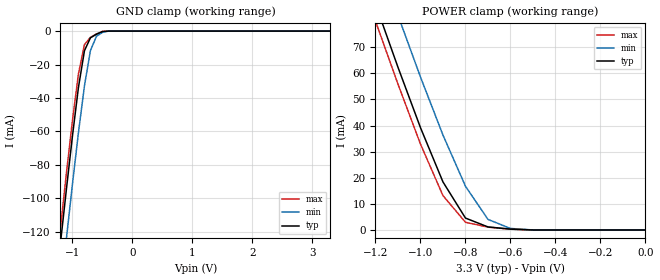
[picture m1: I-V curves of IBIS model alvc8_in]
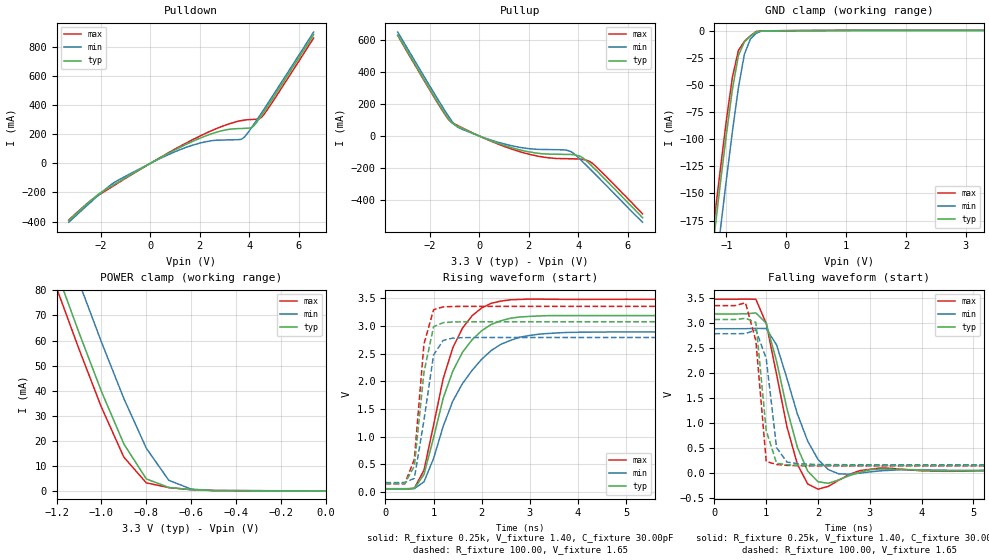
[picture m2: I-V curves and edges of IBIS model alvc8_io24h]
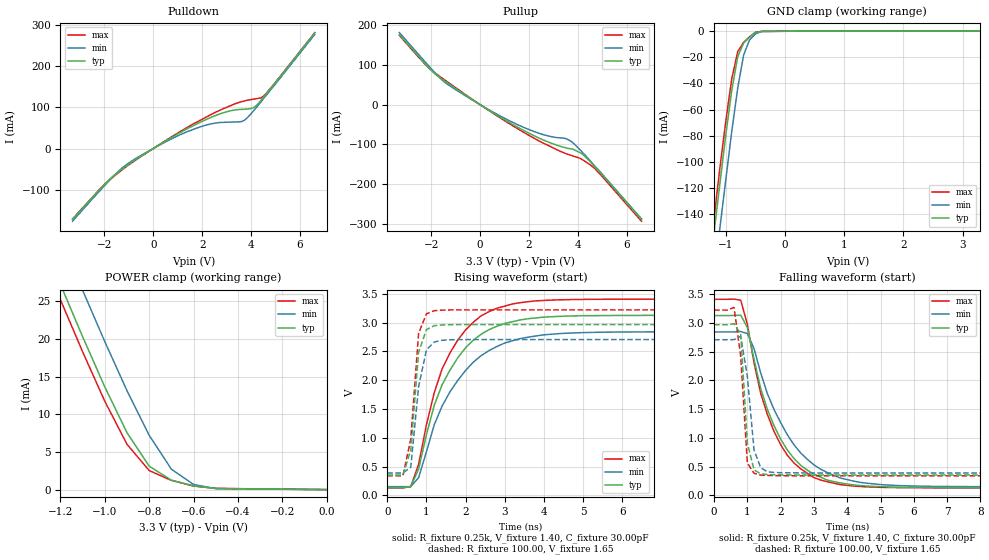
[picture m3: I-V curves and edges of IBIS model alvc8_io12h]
| IBIS file 162245ah.ibs created by s2ibis2 version 1.1
| North Carolina State University Electronics Research Laboratory  1995
[IBIS ver]   2.1
[File name]   162245ah.ibs
[File Rev]   1.0
[Date]   03/01/99 rtk rtk
[Source]   Integrated Device Technology, Inc.
[Notes]   1.Temperatures: typ=25C, min=100C, max=0C 2.RRmp rates based
   on 50 ohm load.
[Disclaimer] Integrated Device Technology, Inc. ("IDT") hereby grants the
   user of this IBIS model a non-exclusive, nontransferable
   license to use this IBIS model under the following terms. The
   user is granted this license only to use the IBIS model and is
   not granted rights to sell, copy (except as needed to run the
   IBIS model), rent, lease or sub-license the IBIS model in
   whole or in part, or in modified form to anyone. The User may
   modify the IBIS model to suit its specific applications, but
   rights to derivative works and such modifications shall belong
   to IDT. This IBIS model is provided on an AS IS" basis and IDT
   makes absolutely no warranty with respect to the information
   contained herein. IDT DISCLAIMS AND CUSTOMER WAIVES ALL
   WARRANTIES, EXPRESS AND IMPLIED, INCLUDING WARRANTIES OF
   MERCHANTABILITY AND FITNESS FOR A PARTICULAR PURPOSE. THE
   ENTIRE RISK AS TO QUALITY AND PERFORMANCE IS WITH THE USER
   ACCORDINGLY, IN NO EVENT SHALL IDT BE LIABLE FOR ANY DIRECT OR
   INDIRECT DAMAGES, WHETHER IN CONTRACT OR TORT, INCLUDING ANY
   LOST PROFITS OR OTHER INCIDENTAL, CONSEQUENTIAL, EXEMPLARY, OR
   PUNITIVE DAMAGES ARISING OUT OF THE USE OR APPLICATION OF THE
   IBIS model. Further, IDT reserves the right to make changes
   without notice to any product herein to improve reliability,
   function, or design. IDT does not convey any license under
   patent rights or any other intellectual property rights,
   including those of third parties. IDT is not obligated to
   provide maintenance or support for the licensed IBIS model.
[Copyright]   Copyright 1997, Integrated Device Technology, Inc. all rights
   reserved
|   Component ALVCH162245
[Component]   ALVCH162245
[Manufacturer]   Integrated Device Technology
[Package]
| PA48
| variable   typ   min   max
R_pkg   6.50m   5.00m   10.00m
L_pkg   3.20nH   2.50nH   4.40nH
C_pkg   0.27pF   0.01pF   0.98pF
| PV48   typ   min   max
|R_pkg   6.5m   5.00m   10.00m
|L_pkg   4.75nH   3.82nH   6.72nH
|C_pkg   0.24pF   0.01pF   1.55pF
[Pin]  signal_name   model_name   R_pin   L_pin   C_pin
1   1DIR   alvc8_in
2   1B1   alvc8_io24h
3   1B2   alvc8_io24h
4   GND   GND
5   1B3   alvc8_io24h
6   1B4   alvc8_io24h
7   VCC   POWER
8   1B5   alvc8_io24h
9   1B6   alvc8_io24h
10   GND   GND
11   1B7   alvc8_io24h
12   1B8   alvc8_io24h
13   2B1   alvc8_io24h
14   2B2   alvc8_io24h
15   GND   GND
16   2B3   alvc8_io24h
17   2B4   alvc8_io24h
18   VCC   POWER
19   2B5   alvc8_io24h
20   2B6   alvc8_io24h
21   GND   GND
22   2B7   alvc8_io24h
23   2B8   alvc8_io24h
24   2DIR   alvc8_in
25   2OEB   alvc8_in
26   2A8   alvc8_io12h
27   2A7   alvc8_io12h
28   GND   GND
29   2A6   alvc8_io12h
30   2A5   alvc8_io12h
31   VCC   POWER
32   2A4   alvc8_io12h
33   2A3   alvc8_io12h
34   GND   GND
35   2A2   alvc8_io12h
36   2A1   alvc8_io12h
37   1A8   alvc8_io12h
38   1A7   alvc8_io12h
39   GND   GND
40   1A6   alvc8_io12h
41   1A5   alvc8_io12h
42   VCC   POWER
43   1A4   alvc8_io12h
44   1A3   alvc8_io12h
45   GND   GND
46   1A2   alvc8_io12h
47   1A1   alvc8_io12h
48   1OEB   alvc8_in
| Models and submodels in the file (3): alvc8_in (Input), alvc8_io24h (I/O), alvc8_io12h (I/O)
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| in   in   dummy_model
| oe   oe   dummy_model
|   Model alvc8_in
[Model]   alvc8_in
Model_type   Input
Vinl =  0.800V
Vinh =  2.000V
C_comp   3.00pF   NA   NA
[Temperature Range]   25.00   100.00   0.000
[Voltage Range]   3.30V   3.00V   3.60V
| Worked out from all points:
|   GND clamp passes 1 mA (typ) near -0.54 V on its own axis
|   POWER clamp passes 1 mA (typ) near -0.68 V on its own axis
[GND_clamp]
| voltage   I(typ)   I(min)   I(max)
-3.3V     -860mA     -887mA     -851mA
-1.3V     -161mA     -190mA     -151mA
-1.2V     -127mA     -157mA     -118mA
-1.1V     -94.41mA   -124mA     -84.85mA
-1V       -62.78mA   -91.54mA   -53.52mA
-900mV    -33.71mA   -60.78mA   -25.6mA
-800mV    -11.74mA   -32.83mA   -8.09mA
-700mV    -4.033mA   -11.65mA   -3.7mA
-600mV    -1.899mA   -3.108mA   -1.699mA
-500mV    -308uA     -810uA     -172uA
-400mV    -3.848nA   -9.872uA   -399pA
3.3V      39.6pA     19.33nA    26.4pA
[POWER_clamp]
| voltage   I(typ)   I(min)   I(max)
-3.3V     630mA      648mA      624mA
-1.2V     86.56mA    106mA      80.02mA
-1.1V     62.33mA    82.22mA    55.88mA
-1V       39.2mA     58.61mA    32.91mA
-900mV    18.4mA     36.35mA    13.15mA
-800mV    4.556mA    16.76mA    2.954mA
-700mV    1.164mA    4.056mA    1.087mA
-600mV    320uA      578uA      299uA
-500mV    40.08nA    12.23uA    3.465nA
0V        39.6pA     59.11pA    43.2pA
|   Model alvc8_io24h
[Model]   alvc8_io24h
Model_type   I/O
Polarity   Non-Inverting
Enable   Active-High
Vinl =  0.000V
Vinh =  2.000V
Vmeas =  1.500V
C_comp   3.00pF   NA   NA
[Temperature Range]   25.00   100.00   0.000
[Voltage Range]   3.30V   3.00V   3.60V
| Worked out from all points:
|   slope of the pulldown table from 0 to 0.495 V, typ, clamps not added: 10.5 ohm
|   slope of the pullup table from 0 to 0.495 V, typ, clamps not added: 16.1 ohm
|   GND clamp passes 1 mA (typ) near -0.50 V on its own axis
|   POWER clamp passes 1 mA (typ) near -0.66 V on its own axis
|   rising waveform, R_fixture 0.25k, V_fixture 1.40, C_fixture 30.00pF: 20-80 % time 723ps typ, 920ps min, 623ps max; typ from 0.055 V to 3.19 V
|   rising waveform, R_fixture 100.00, V_fixture 1.65: 20-80 % time 248ps typ, 279ps min, 194ps max; typ from 0.155 V to 3.08 V
|   falling waveform, R_fixture 0.25k, V_fixture 1.40, C_fixture 30.00pF: 20-80 % time 444ps typ, 538ps min, 413ps max; typ from 3.19 V to 0.055 V
|   falling waveform, R_fixture 100.00, V_fixture 1.65: 20-80 % time 187ps typ, 176ps min, 171ps max; typ from 3.08 V to 0.155 V
[Pulldown]
| voltage   I(typ)   I(min)   I(max)
-3.3V     -392mA     -404mA     -389mA
-2.3V     -240mA     -249mA     -241mA
-1.5V     -149mA     -136mA     -156mA
300mV     28.8mA     25.5mA     30.3mA
1.4V      127mA      107mA      135mA
2.4V      199mA      153mA      219mA
3.6V      239mA      163mA      291mA
3.8V      240mA      180mA      297mA
4.2V      260mA      272mA      302mA
4.4V      306mA      322mA      306mA
4.6V      356mA      373mA      337mA
6.6V      883mA      901mA      860mA
[Pullup]
| voltage   I(typ)   I(min)   I(max)
-3.3V     630mA      649mA      628mA
-1.4V     142mA      160mA      137mA
-1.1V     80.6mA     90.7mA     83.6mA
-900mV    63mA       57.7mA     67.6mA
400mV     -25.1mA    -21.5mA    -27.4mA
1.6V      -85mA      -69.5mA    -95.9mA
2.6V      -111mA     -84mA      -132mA
3.4V      -115mA     -86.1mA    -141mA
3.7V      -115mA     -97.1mA    -142mA
4.1V      -128mA     -149mA     -144mA
4.5V      -179mA     -210mA     -162mA
6.6V      -510mA     -538mA     -486mA
[GND_clamp]
| voltage   I(typ)   I(min)   I(max)
-3.3V     -1.238A    -1.278A    -1.225A
-1.3V     -235mA     -278mA     -221mA
-1.2V     -187mA     -230mA     -173mA
-1.1V     -140mA     -183mA     -127mA
-1V       -95.39mA   -137mA     -82.2mA
-900mV    -54.08mA   -92.95mA   -42.96mA
-800mV    -22.96mA   -52.74mA   -18.28mA
-700mV    -10.43mA   -21.77mA   -9.816mA
-600mV    -5.251mA   -7.746mA   -4.745mA
-500mV    -1.015mA   -2.281mA   -688uA
-400mV    -144uA     -128uA     -169uA
3.3V      264uA      161uA      341uA
[POWER_clamp]
| voltage   I(typ)   I(min)   I(max)
-3.3V     638mA      656mA      632mA
-1.2V     87.67mA    108mA      81.05mA
-1.1V     63.19mA    83.28mA    56.62mA
-1V       39.75mA    59.43mA    33.41mA
-900mV    18.73mA    36.86mA    13.47mA
-800mV    4.8mA      17.05mA    3.222mA
-700mV    1.374mA    4.243mA    1.32mA
-600mV    498uA      728uA      497uA
-500mV    146uA      134uA      162uA
0V        111pA      156pA      121pA
[Ramp]
| variable   typ   min   max
dV/dt_r   1.48/0.31n   1.29/0.30n   1.66/0.22n
dV/dt_f   1.63/0.28n   1.45/0.31n   1.80/0.19n
R_load = 50.00
[Rising Waveform]
R_fixture = 0.25k
V_fixture = 1.40
C_fixture = 30.00pF
R_dut = 7.00m
L_dut = 3.30nH
C_dut = 0.29pF
| time   V(typ)   V(min)   V(max)
0s        55.43mV    62mV       53.03mV
600ps     66.6mV     63.52mV    70.73mV
800ps     318mV      185mV      393mV
1ns       982mV      608mV      1.211V
1.2ns     1.697V     1.189V     2.05V
1.4ns     2.186V     1.644V     2.606V
1.8ns     2.751V     2.198V     3.185V
2.4ns     3.095V     2.67V      3.451V
3.8ns     3.189V     2.885V     3.481V
19.8ns    3.189V     2.893V     3.482V
[Rising Waveform]
R_fixture = 100.00
V_fixture = 1.65
R_dut = 7.00m
L_dut = 3.30nH
C_dut = 0.29pF
| time   V(typ)   V(min)   V(max)
0s        155mV      172mV      148mV
400ps     155mV      173mV      148mV
600ps     469mV      249mV      594mV
800ps     2.166V     1.299V     2.675V
1ns       2.988V     2.477V     3.294V
1.2ns     3.061V     2.741V     3.346V
1.4ns     3.073V     2.782V     3.353V
2ns       3.077V     2.793V     3.355V
19.8ns    3.077V     2.793V     3.355V
[Falling Waveform]
R_fixture = 0.25k
V_fixture = 1.40
C_fixture = 30.00pF
R_dut = 7.00m
L_dut = 3.30nH
C_dut = 0.29pF
| time   V(typ)   V(min)   V(max)
0s        3.189V     2.893V     3.482V
800ps     3.208V     2.901V     3.481V
1ns       3.002V     2.896V     2.998V
1.2ns     2.239V     2.568V     1.977V
1.4ns     1.294V     1.899V     934mV
1.6ns     525mV      1.193V     186mV
2ns       -168mV     277mV      -316mV
2.4ns     -131mV     -10.2mV    -138mV
3.2ns     86.4mV     50.55mV    107mV
19.8ns    55.43mV    62mV       53.03mV
[Falling Waveform]
R_fixture = 100.00
V_fixture = 1.65
R_dut = 7.00m
L_dut = 3.30nH
C_dut = 0.29pF
| time   V(typ)   V(min)   V(max)
0s        3.077V     2.793V     3.355V
400ps     3.077V     2.793V     3.355V
600ps     3.101V     2.795V     3.411V
800ps     3.02V      2.869V     2.651V
1ns       857mV      2.294V     237mV
1.2ns     202mV      512mV      177mV
1.4ns     172mV      227mV      160mV
1.6ns     163mV      194mV      154mV
2ns       157mV      178mV      149mV
19.8ns    155mV      172mV      148mV
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|   Model alvc8_io12h
[Model]   alvc8_io12h
Model_type   I/O
Polarity   Non-Inverting
Enable   Active-High
Vinl =  0.000V
Vinh =  2.000V
Vmeas =  1.500V
C_comp   3.00pF   NA   NA
[Temperature Range]   25.00   100.00   0.000
[Voltage Range]   3.30V   3.00V   3.60V
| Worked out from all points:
|   slope of the pulldown table from 0 to 0.495 V, typ, clamps not added: 27.5 ohm
|   slope of the pullup table from 0 to 0.495 V, typ, clamps not added: 25.8 ohm
|   GND clamp passes 1 mA (typ) near -0.50 V on its own axis
|   POWER clamp passes 1 mA (typ) near -0.67 V on its own axis
|   rising waveform, R_fixture 0.25k, V_fixture 1.40, C_fixture 30.00pF: 20-80 % time 1.07ns typ, 1.21ns min, 991ps max; typ from 0.137 V to 3.12 V
|   rising waveform, R_fixture 100.00, V_fixture 1.65: 20-80 % time 184ps typ, 259ps min, 200ps max; typ from 0.354 V to 2.96 V
|   falling waveform, R_fixture 0.25k, V_fixture 1.40, C_fixture 30.00pF: 20-80 % time 1.13ns typ, 1.37ns min, 1.04ns max; typ from 3.12 V to 0.137 V
|   falling waveform, R_fixture 100.00, V_fixture 1.65: 20-80 % time 176ps typ, 241ps min, 216ps max; typ from 2.96 V to 0.354 V
[Pulldown]
| voltage   I(typ)   I(min)   I(max)
-3.3V     -172mA     -177mA     -171mA
-1.8V     -76mA      -78.1mA    -76.9mA
-1.3V     -51.4mA    -48.7mA    -53mA
-700mV    -26.3mA    -23.6mA    -27.4mA
800mV     28.7mA     25.1mA     30.3mA
1.8V      60.3mA     50.2mA     64.7mA
2.9V      87.5mA     63.7mA     97.9mA
3.7V      95.5mA     67.7mA     115mA
4.1V      99.3mA     91.8mA     120mA
4.5V      124mA      121mA      127mA
5V        161mA      157mA      161mA
6.6V      281mA      277mA      282mA
[Pullup]
| voltage   I(typ)   I(min)   I(max)
-3.3V     176mA      181mA      174mA
-1.9V     80.3mA     83.6mA     82mA
-1.5V     61.8mA     58.9mA     64.3mA
-1V       40.8mA     37.7mA     42.5mA
400mV     -15.6mA    -14.2mA    -16.4mA
1.7V      -62.2mA    -54.9mA    -66.6mA
2.9V      -96.6mA    -80.2mA    -106mA
3.5V      -108mA     -85.3mA    -123mA
3.8V      -112mA     -96mA      -129mA
4.2V      -125mA     -121mA     -139mA
4.7V      -156mA     -155mA     -161mA
6.6V      -289mA     -287mA     -293mA
[GND_clamp]
| voltage   I(typ)   I(min)   I(max)
-3.3V     -1.019A    -1.052A    -1.008A
-1.3V     -194mA     -229mA     -182mA
-1.2V     -154mA     -189mA     -143mA
-1.1V     -116mA     -150mA     -104mA
-1V       -78.66mA   -113mA     -68.13mA
-900mV    -44.91mA   -76.33mA   -36.12mA
-800mV    -19.38mA   -43.36mA   -15.48mA
-700mV    -9.002mA   -18.09mA   -8.455mA
-600mV    -4.636mA   -6.615mA   -4.212mA
-500mV    -941uA     -2.052mA   -652uA
-400mV    -144uA     -128uA     -169uA
3.3V      264uA      161uA      341uA
[POWER_clamp]
| voltage   I(typ)   I(min)   I(max)
-3.3V     183mA      189mA      181mA
-1.3V     34.33mA    40.55mA    32.29mA
-1.2V     27.22mA    33.44mA    25.19mA
-1.1V     20.28mA    26.44mA    18.28mA
-1V       13.61mA    19.62mA    11.71mA
-900mV    7.542mA    13.11mA    6.005mA
-800mV    3.103mA    7.194mA    2.527mA
-700mV    1.249mA    2.702mA    1.219mA
-600mV    484uA      674uA      476uA
-500mV    146uA      134uA      162uA
0V        111pA      156pA      121pA
[Ramp]
| variable   typ   min   max
dV/dt_r   1.29/0.24n   1.13/0.30n   1.44/0.25n
dV/dt_f   1.26/0.26n   1.08/0.26n   1.40/0.24n
R_load = 50.00
[Rising Waveform]
R_fixture = 0.25k
V_fixture = 1.40
C_fixture = 30.00pF
R_dut = 7.00m
L_dut = 3.30nH
C_dut = 0.29pF
| time   V(typ)   V(min)   V(max)
0s        137mV      152mV      131mV
600ps     152mV      153mV      153mV
800ps     459mV      307mV      538mV
1.2ns     1.566V     1.227V     1.783V
1.4ns     1.921V     1.551V     2.196V
1.8ns     2.389V     1.996V     2.696V
2.4ns     2.799V     2.427V     3.119V
3.2ns     3.016V     2.685V     3.324V
5.6ns     3.122V     2.834V     3.405V
19.8ns    3.125V     2.84V      3.407V
[Rising Waveform]
R_fixture = 100.00
V_fixture = 1.65
R_dut = 7.00m
L_dut = 3.30nH
C_dut = 0.29pF
| time   V(typ)   V(min)   V(max)
0s        354mV      389mV      341mV
400ps     354mV      390mV      341mV
600ps     788mV      488mV      976mV
800ps     2.487V     1.886V     2.814V
1ns       2.877V     2.527V     3.153V
1.2ns     2.947V     2.663V     3.206V
1.4ns     2.959V     2.693V     3.216V
2ns       2.965V     2.705V     3.22V
19.8ns    2.965V     2.705V     3.22V
[Falling Waveform]
R_fixture = 0.25k
V_fixture = 1.40
C_fixture = 30.00pF
R_dut = 7.00m
L_dut = 3.30nH
C_dut = 0.29pF
| time   V(typ)   V(min)   V(max)
0s        3.125V     2.84V      3.407V
800ps     3.131V     2.846V     3.392V
1ns       2.917V     2.813V     2.972V
1.4ns     1.855V     2.128V     1.774V
1.8ns     1.213V     1.493V     1.113V
2.4ns     640mV      880mV      563mV
3.2ns     318mV      456mV      267mV
4.2ns     181mV      247mV      162mV
5.6ns     143mV      169mV      135mV
19.8ns    137mV      152mV      131mV
[Falling Waveform]
R_fixture = 100.00
V_fixture = 1.65
R_dut = 7.00m
L_dut = 3.30nH
C_dut = 0.29pF
| time   V(typ)   V(min)   V(max)
0s        2.965V     2.705V     3.22V
400ps     2.965V     2.705V     3.22V
600ps     2.984V     2.706V     3.266V
800ps     2.805V     2.763V     2.411V
1ns       908mV      2.064V     561mV
1.2ns     444mV      789mV      384mV
1.4ns     374mV      481mV      353mV
1.6ns     362mV      411mV      347mV
2ns       357mV      394mV      343mV
19.8ns    354mV      389mV      341mV
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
